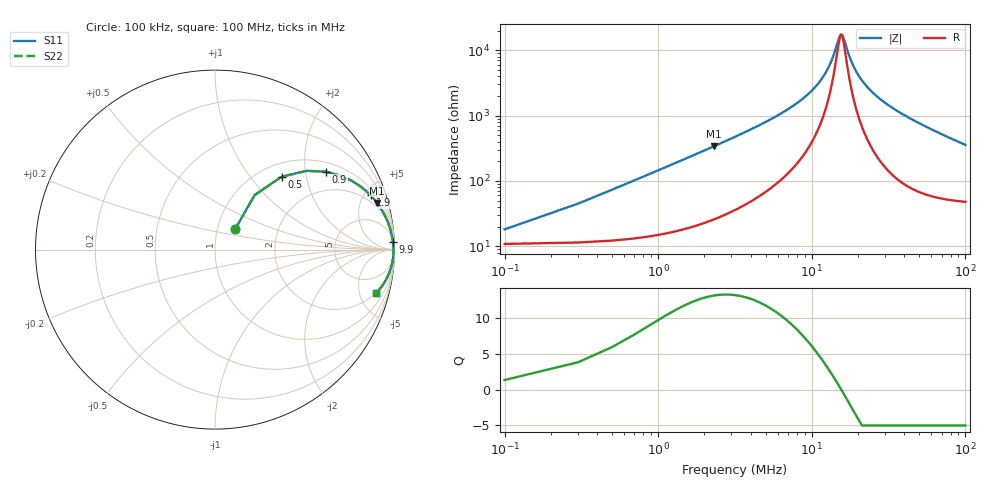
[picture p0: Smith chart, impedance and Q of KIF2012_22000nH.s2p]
!version-2
!date-12.2020
!Series
# MHz S RI R 50
!Freq ReS11 ImS11 ReS21 ImS21 ReS12 ImS12 ReS22 ImS22
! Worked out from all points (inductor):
!   501 points, 100 kHz to 100 MHz, reference 50 ohm
!   read as one part in series: L = 23 uH near 500 kHz
!   highest Q = 13.1 at 2.3 MHz (marker M1), where L = 23.4 uH
!   self-resonance near 15.5 MHz
!   S11 on the Smith chart (normalised r, x): 100 kHz: 1.22, +0.29; 500 kHz: 1.24, +1.45; 900 kHz: 1.29, +2.61; 1.9 MHz: 1.44, +5.55; 9.9 MHz: 9, +47; 100 MHz: 1.96, -7.07
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0.1  0.1133 0.1163  0.8867 -0.1163  0.8867 -0.1163  0.1133 0.1163
0.5  0.3706 0.4058  0.6294 -0.4058  0.6294 -0.4058  0.3706 0.4058
0.7  0.5093 0.439  0.4907 -0.439  0.4907 -0.439  0.5093 0.439
0.9  0.6194 0.4337  0.3806 -0.4337  0.3806 -0.4337  0.6194 0.4337
1.3  0.7624 0.383  0.2376 -0.383  0.2376 -0.383  0.7624 0.383
1.9  0.8672 0.3022  0.1328 -0.3022  0.1328 -0.3022  0.8672 0.3022
2.3  0.9032 0.26  0.0968 -0.26  0.0968 -0.26  0.9032 0.26
4.7  0.9718 0.1291  0.0282 -0.1291  0.0282 -0.1291  0.9718 0.1291
9.9  0.9916 0.0412  0.00844 -0.0412  0.00844 -0.0412  0.9916 0.0412
12.7  0.9937 0.018  0.00635 -0.018  0.00635 -0.018  0.9937 0.018
15.3  0.9943 0.00142  0.0057 -0.00142  0.0057 -0.00142  0.9943 0.00142
15.9  0.9943 -0.00199  0.00566 0.00199  0.00566 0.00199  0.9943 -0.00199
16.9  0.9943 -0.00741  0.00565 0.00741  0.00565 0.00741  0.9943 -0.00741
17.9  0.9943 -0.0125  0.00573 0.0125  0.00573 0.0125  0.9943 -0.0125
19.1  0.9941 -0.0184  0.0059 0.0184  0.0059 0.0184  0.9941 -0.0184
22.3  0.9933 -0.0327  0.00674 0.0327  0.00674 0.0327  0.9933 -0.0327
26.9  0.9913 -0.0509  0.0087 0.0509  0.0087 0.0509  0.9913 -0.0509
33.5  0.9873 -0.0743  0.0127 0.0743  0.0127 0.0743  0.9873 -0.0743
50.1  0.9724 -0.1253  0.0276 0.1253  0.0276 0.1253  0.9724 -0.1253
66.7  0.952 -0.1693  0.048 0.1693  0.048 0.1693  0.952 -0.1693
83.5  0.9269 -0.208  0.0731 0.208  0.0731 0.208  0.9269 -0.208
100  0.8992 -0.2407  0.1008 0.2407  0.1008 0.2407  0.8992 -0.2407
